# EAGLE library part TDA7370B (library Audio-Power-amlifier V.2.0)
The TDA7370B is a new technology class AB quad channels Audio Power Amplifier in Multiwatt package designed for car radio applications. Thanks to the fully complementary PNP/NPN output configuration the high power performances of the TDA7370B are obtained without bootstrap capacitors.
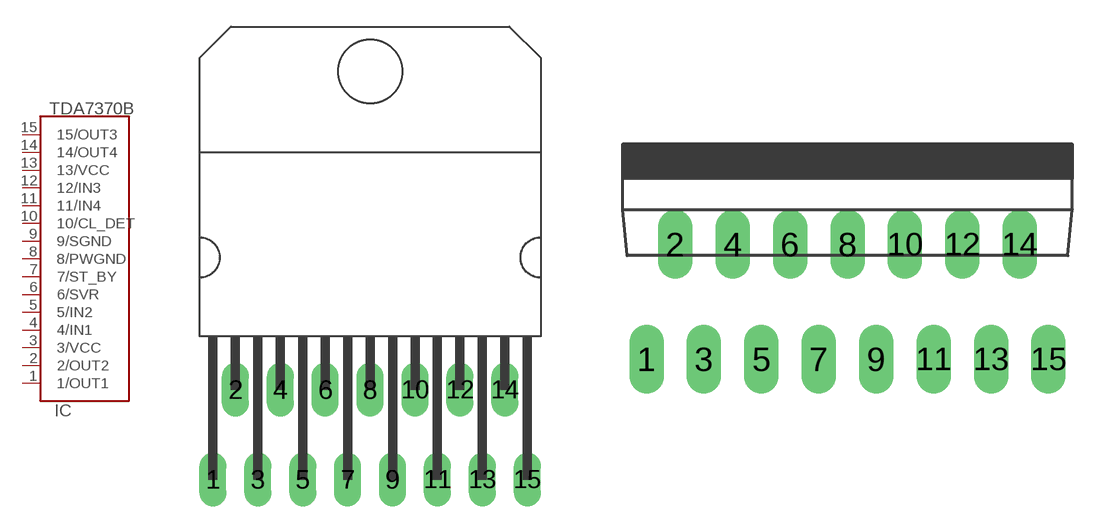
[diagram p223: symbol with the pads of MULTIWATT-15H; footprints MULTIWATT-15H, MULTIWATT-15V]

Designator prefix IC

## TDA7370BH  [MULTIWATT-15H]
1  1/OUT1  out
2  2/OUT2  out
3  3/VCC  pwr
4  4/IN1  in
5  5/IN2  in
6  6/SVR  in
7  7/ST_BY  in
8  8/PWGND  pwr
9  9/SGND  pwr
10  10/CL_DET
11  11/IN4  in
12  12/IN3  in
13  13/VCC  pwr
14  14/OUT4  out
15  15/OUT3  out

## TDA7370BV  [MULTIWATT-15V]
Pads as for MULTIWATT-15H

## Footprint MULTIWATT-15H (pad centres in mm)
Multiwatt 15 horizontal
drill 1.016 long: 1 -8.89,-5.08; 2 -7.62,0; 3 -6.35,-5.08; 4 -5.08,0; 5 -3.81,-5.08; 6 -2.54,0; 7 -1.27,-5.08; 8 0,0; 9 1.27,-5.08; 10 2.54,0; 11 3.81,-5.08; 12 5.08,0; 13 6.35,-5.08; 14 7.62,0; 15 8.89,-5.08

## Footprint MULTIWATT-15V (pad centres in mm)
Multiwatt 15 vertical
drill 1.016 long: 1 -8.89,-5.08; 2 -7.62,0; 3 -6.35,-5.08; 4 -5.08,0; 5 -3.81,-5.08; 6 -2.54,0; 7 -1.27,-5.08; 8 0,0; 9 1.27,-5.08; 10 2.54,0; 11 3.81,-5.08; 12 5.08,0; 13 6.35,-5.08; 14 7.62,0; 15 8.89,-5.08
